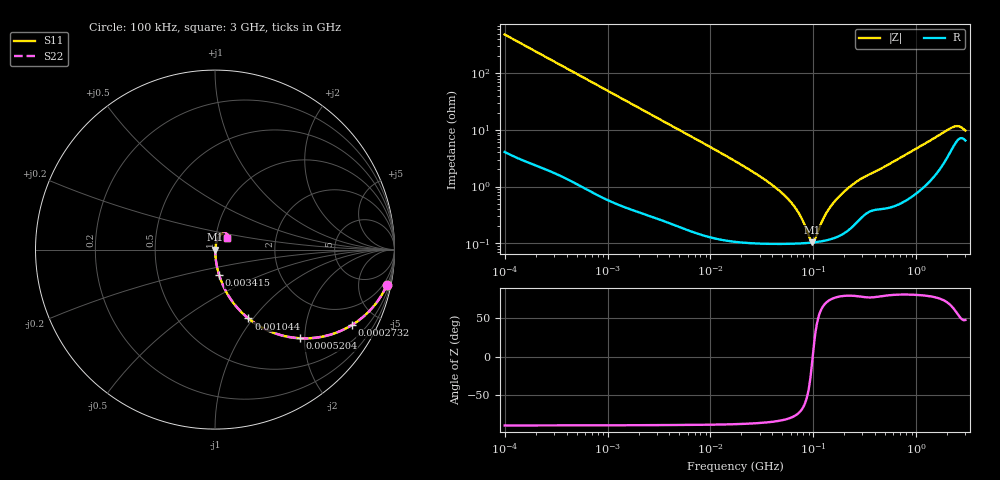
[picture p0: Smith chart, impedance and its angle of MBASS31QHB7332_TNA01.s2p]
! MBASS31QHB7332_TNA01  S-PARAMETER MODEL  ( Standard Model )
! Model Generated by TAIYO YUDEN Corporation (http://www.ty-top.com)
! Version 1.0
! TAIYO YUDEN Control No. 220601
! Copyright(c) 2013 TAIYO YUDEN CO.,LTD. All Rights Reserved.
! Product Description (link to TY-COMPAS)
! https://ds.yuden.co.jp/TYCOMPAS/or/detail?pn=MBASS31QHB7332KTNA01&u=M
! Products Name : Multilayer Ceramic Capacitors
! Characteristics :
!  Capacitance : 3300 [pF] , Rated Voltage : 630 [V] , TCC : X7R
!  Case Size : 3.2 x 1.6 / 0.126 x 0.063 [mm/inch] , Thickness : 1.15 / 0.045 [mm/inch]
!  (Conditions: Temperature = 25 [degC] , DC Bias Voltage = 0 [V])
! External Node Assignments :
!  1  o---| |---o  2
! GND o---------o GND
! Frequency Range : 100kHz  -  3GHz  [ 401 STEP ]
# MHZ S RI R 50
! Freq[MHz].  S11 Real  S11 Imag  S21 Real  S21 Imag  S12 Real  S12 Imag  S22 Real  S22 Imag
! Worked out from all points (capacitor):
!   401 points, 100 kHz to 3 GHz, reference 50 ohm
!   read as one part in series: C = 3.26 nF near 105.3 kHz
!   lowest |Z| = 103 mohm at 97.38 MHz (marker M1)
!   series resonance near 98.47 MHz, so ESL is about 800 pH
!   S11 on the Smith chart (normalised r, x): 100 kHz: 1.08, -9.75; 273.2 kHz: 1.04, -3.59; 520.4 kHz: 1.02, -1.89; 1.044 MHz: 1.01, -0.95; 3.415 MHz: 1.00, -0.29; 3 GHz: 1.13, +0.14
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0.1  0.9581 -0.1962  0.0419 0.1962  0.0419 0.1962  0.9581 -0.1962
0.17181  0.8877 -0.3111  0.1123 0.3111  0.1123 0.3111  0.8877 -0.3111
0.273224  0.7606 -0.4215  0.2394 0.4215  0.2394 0.4215  0.7606 -0.4215
0.520403  0.4728 -0.4937  0.5272 0.4937  0.5272 0.4937  0.4728 -0.4937
0.562235  0.4352 -0.4902  0.5648 0.4902  0.5648 0.4902  0.4352 -0.4902
1.043626  0.1863 -0.3835  0.8137 0.3835  0.8137 0.3835  0.1863 -0.3835
1.702975  0.0812 -0.2665  0.9188 0.2665  0.9188 0.2665  0.0812 -0.2665
3.161081  0.0266 -0.1529  0.9734 0.1529  0.9734 0.1529  0.0266 -0.1529
3.415183  0.0232 -0.1421  0.9768 0.1421  0.9768 0.1421  0.0232 -0.1421
17.7727  0.00179 -0.0273  0.9982 0.0273  0.9982 0.0273  0.00179 -0.0273
35.64176  0.00112 -0.0123  0.9989 0.0123  0.9989 0.0123  0.00112 -0.0123
55.23785  0.00101 -0.00625  0.999 0.00625  0.999 0.00625  0.00101 -0.00625
73.34282  0.000993 -0.00306  0.999 0.00306  0.999 0.00306  0.000993 -0.00306
97.38194  0.00102 -0.000114  0.999 0.000114  0.999 0.000114  0.00102 -0.000114
105.21  0.00104 0.000682  0.999 -0.000682  0.999 -0.000682  0.00104 0.000682
136.1397  0.00114 0.00341  0.9989 -0.00341  0.9989 -0.00341  0.00114 0.00341
180.7614  0.00139 0.00672  0.9986 -0.00672  0.9986 -0.00672  0.00139 0.00672
280.1453  0.00274 0.0128  0.9973 -0.0128  0.9973 -0.0128  0.00274 0.0128
547.5153  0.0048 0.0244  0.9952 -0.0244  0.9952 -0.0244  0.0048 0.0244
2145.926  0.0479 0.0905  0.9521 -0.0905  0.9521 -0.0905  0.0479 0.0905
2504.792  0.0686 0.0851  0.9314 -0.0851  0.9314 -0.0851  0.0686 0.0851
3000  0.0655 0.0635  0.9345 -0.0635  0.9345 -0.0635  0.0655 0.0635
